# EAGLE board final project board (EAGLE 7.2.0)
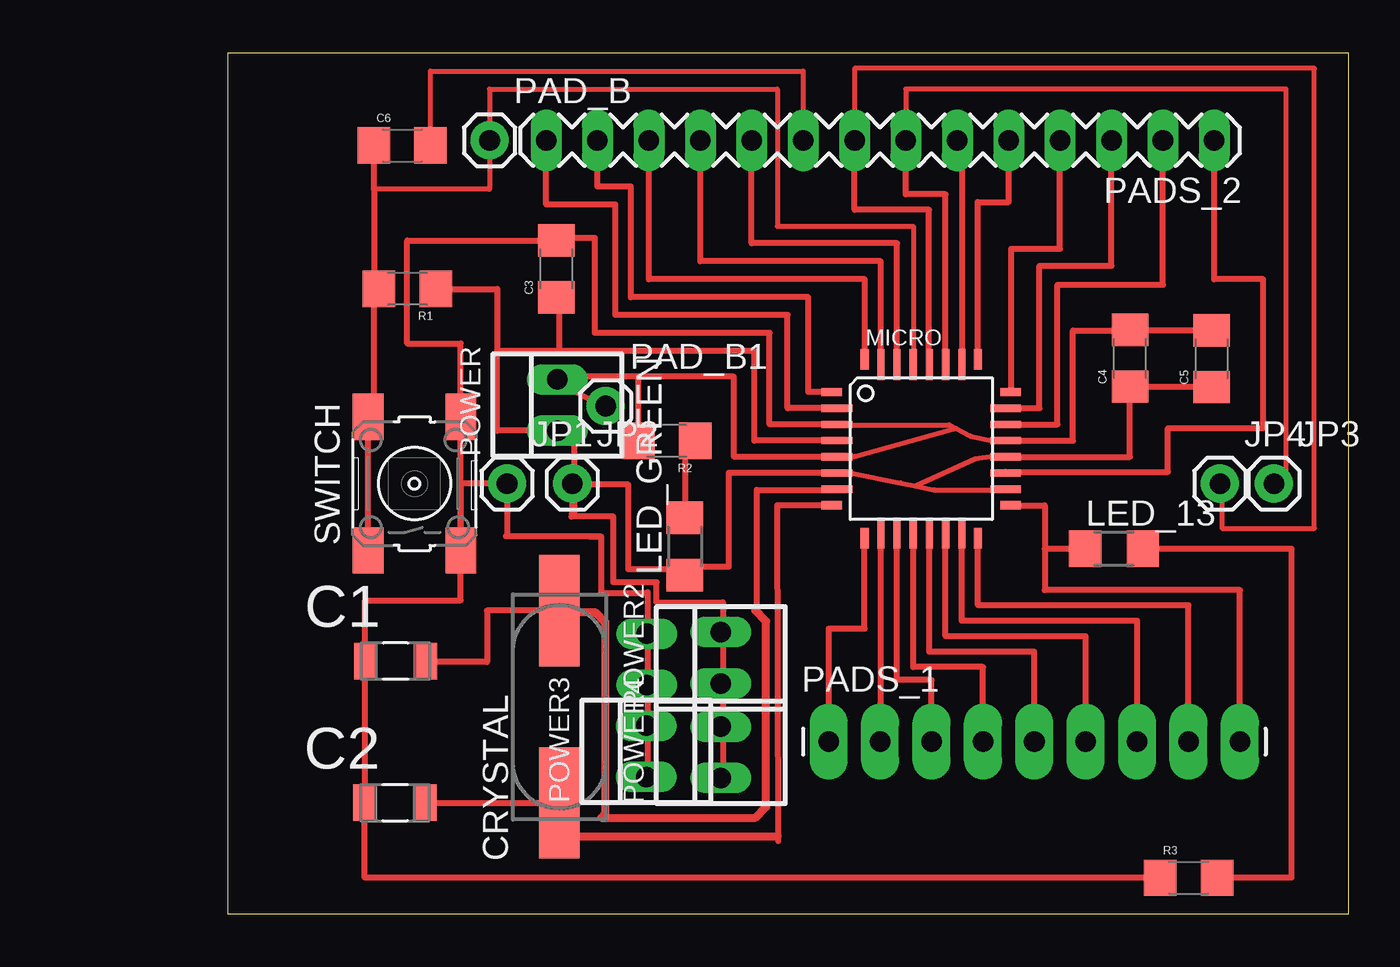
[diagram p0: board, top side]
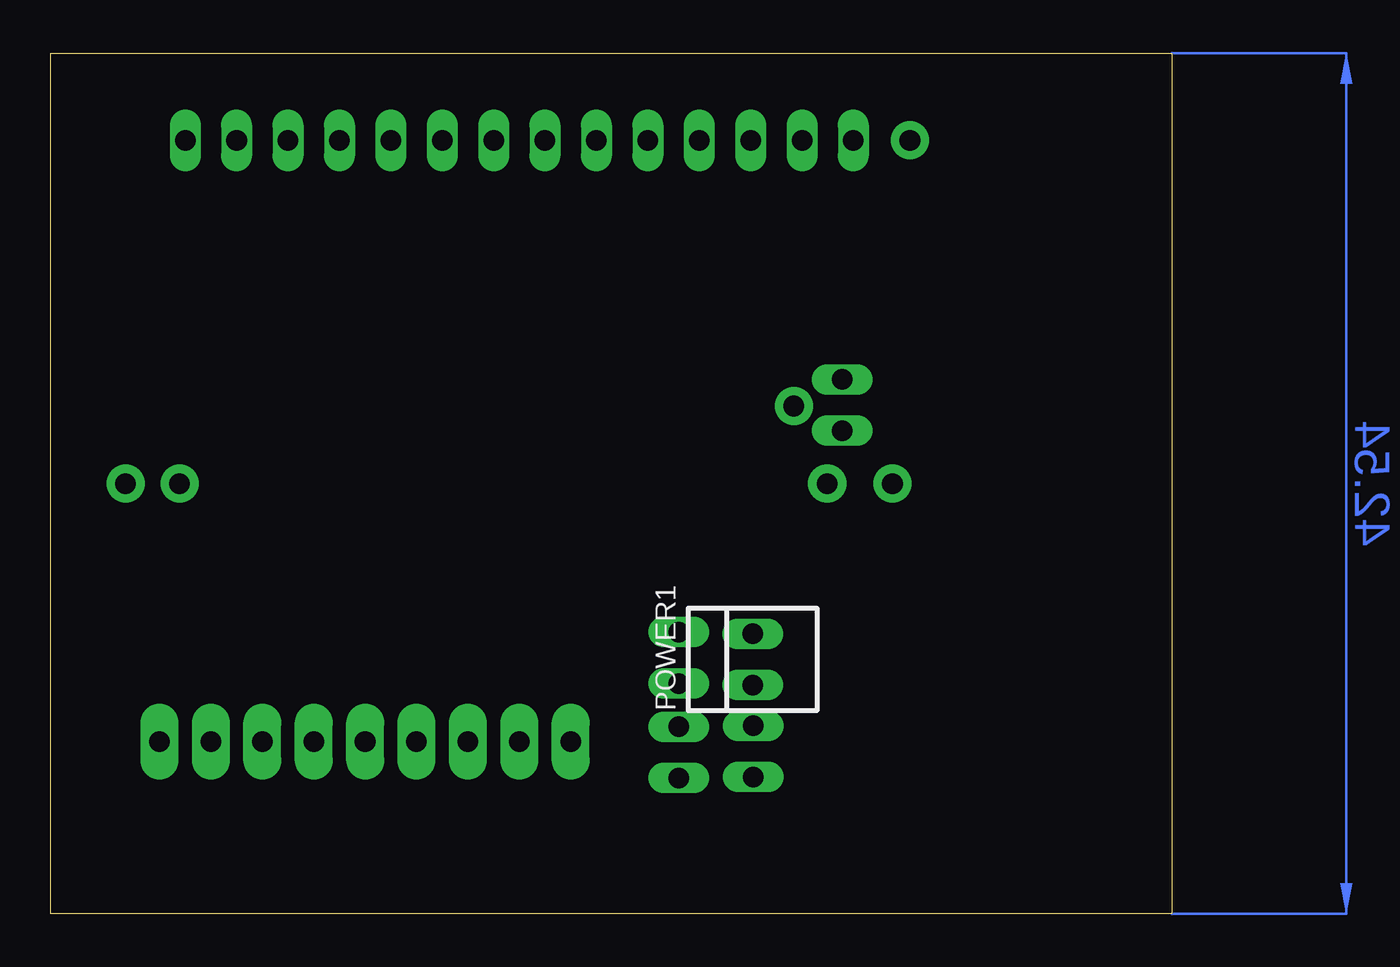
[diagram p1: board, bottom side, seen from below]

Size 55.42 x 42.54 mm. Coordinates in mm from the lower left corner, seen from the top.
Outline: 0,0 55.42,0 55.42,42.54 0,42.54 0,0
Copper layers (1*16): Top 0.035mm / dielectric 1.5mm / Bottom 0.035mm
Design rules "default": minimum track width 10mil, minimum drill 24mil, track to track 8mil, track to pad 8mil, pad to pad 8mil, via to via 8mil, smd to smd 8mil, copper to edge 40mil, drill to drill 8mil, minimum pad ring 10mil, minimum via ring 8mil, stop-mask expansion 4mil, vias tented up to drill 0mil, thermal gap 10mil

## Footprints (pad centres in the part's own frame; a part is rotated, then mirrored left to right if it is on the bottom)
CAPC3216X178N = smd 1.118 x 1.803: 1 -1.499,0; 2 1.499,0
1206 = smd 1.6 x 1.8: 1 -1.4,0; 2 1.4,0
CSM-7X-DU = smd 5.5 x 2: 1 -4.75,0; 2 4.75,0
1X01 = drill 1.016 pad 1.88: 1 0,0
1206' = smd 1.6 x 1.803: 1 -1.422,0; 2 1.422,0
TQFP32-08 = smd 1.016 x 0.406: 1 -4.42,2.8; 8 -4.42,-2.8; 17 4.42,-2.8; 24 4.42,2.8 | smd 1.524 x 0.356: 2 -4.166,2; 3 -4.166,1.2; 4 -4.166,0.4; 5 -4.166,-0.4; 6 -4.166,-1.2; 7 -4.166,-2; 18 4.166,-2; 19 4.166,-1.2; 20 4.166,-0.4; 21 4.166,0.4; 22 4.166,1.2; 23 4.166,2 | smd 0.406 x 1.016: 9 -2.8,-4.42; 16 2.8,-4.42; 25 2.8,4.42; 32 -2.8,4.42 | smd 0.356 x 1.524: 10 -2,-4.166; 11 -1.2,-4.166; 12 -0.4,-4.166; 13 0.4,-4.166; 14 1.2,-4.166; 15 2,-4.166; 26 2,4.166; 27 1.2,4.166; 28 0.4,4.166; 29 -0.4,4.166; 30 -1.2,4.166; 31 -2,4.166
1X09_LONGPADS = drill 1.016 pad 1.88 long: 1 0,0; 2 2.54,0; 3 5.08,0; 4 7.62,0; 5 10.16,0; 6 12.7,0; 7 15.24,0; 8 17.78,0; 9 20.32,0
1X14-LONGPADS = drill 1.016 long: 1 0,0; 2 2.54,0; 3 5.08,0; 4 7.62,0; 5 10.16,0; 6 12.7,0; 7 15.24,0; 8 17.78,0; 9 20.32,0; 10 22.86,0; 11 25.4,0; 12 27.94,0; 13 30.48,0; 14 33.02,0
22-23-2021 = drill 1 long: 1 -1.27,0; 2 1.27,0
6MM_SWITCH = smd 2.286 x 1.524: 1 -3.302,2.286; 2 3.302,2.286; 3 -3.302,-2.286; 4 3.302,-2.286

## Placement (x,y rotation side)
C1  22pF  [CAPC3216X178N]  8.31,12.5 0 top
C2  22pF  [CAPC3216X178N]  8.28,5.49 0 top
C3  10uF  [1206]  16.26,31.88 90 top
C4  1uF  [1206]  44.6,27.46 90 top
C5  100nF  [1206]  48.64,27.43 90 top
C6  100nF  [1206]  8.64,37.97 0 top
CRYSTAL  16Mhz  [CSM-7X-DU]  16.41,10.24 90 top
JP1  M01PTH  [1X01]  13.82,21.26 0 top
JP2  M01PTH  [1X01]  17.04,21.26 0 top
JP3  M01PTH  [1X01]  51.71,21.26 0 top
JP4  M01PTH  [1X01]  49.05,21.26 0 top
LED_13  YELLOW  [1206']  43.81,18.03 0 top
LED_GREEN  [1206']  22.61,18.16 90 top
MICRO  ATMEGA328P-AU  [TQFP32-08]  34.29,22.99 0 top
PAD_B  M01PTH  [1X01]  12.95,38.23 0 top
PAD_B1  M01PTH  [1X01]  18.69,25.1 0 top
PADS_1  M09LONGPADS  [1X09_LONGPADS]  29.72,8.51 0 top
PADS_2  M14LONGPADS  [1X14-LONGPADS]  48.77,38.23 180 top
POWER  22-23-2021  [22-23-2021]  16.31,25.15 90 top
POWER1  22-23-2021  [22-23-2021]  20.73,12.57 90 bottom
POWER2  22-23-2021  [22-23-2021]  24.38,12.65 90 top
POWER3  22-23-2021  [22-23-2021]  20.7,8.03 90 top
POWER4  22-23-2021  [22-23-2021]  24.38,7.98 90 top
R1  10k  [1206]  8.89,30.89 180 top
R2  499  [1206]  21.72,23.37 180 top
R3  499  [1206]  47.5,1.78 0 top
SWITCH  [6MM_SWITCH]  9.25,21.26 90 top

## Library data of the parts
C1 C2 = AVX_By_element14_Batch_1; MPN: 0612ZC225MAT2A; OC_FARNELL: -; OC_NEWARK: 12N3209; SUPPLIER: AVX; TOLERANCE: ±20%; VOLTAGERATING: 10V
C3-C6 JP1-JP4 PAD_B PAD_B1 PADS_1 PADS_2 R1-R3 = 01_SparkFun
CRYSTAL = 01_FAB_Hello; OC_FARNELL: unknown; OC_NEWARK: unknown
LED_13 LED_GREEN SWITCH = 01_FAB_Hello
MICRO = atmega8
POWER POWER1-POWER4 = con-molex; MF: MOLEX; MPN: 22-23-2021; OC_FARNELL: 1462926; OC_NEWARK: 25C3832

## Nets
GND: C1.1 C2.1 C3.2 C4.2 C5.2 JP1.1 MICRO.3 MICRO.5 MICRO.21 POWER.2 R2.2 R3.1 SWITCH.3 SWITCH.4
N$1: MICRO.9 PADS_1.1
N$2: MICRO.7
N$3: C6.2 PADS_2.9
N$4: MICRO.10 PADS_1.2
N$5: MICRO.11 PADS_1.3
N$6: MICRO.12 PADS_1.4
N$7: MICRO.13 PADS_1.5
N$8: MICRO.14 PADS_1.6
N$9: MICRO.8
N$10: MICRO.15 PADS_1.7
N$11: MICRO.16 PADS_1.8
N$12: LED_13.1 MICRO.17 PADS_1.9
N$13: MICRO.19 PADS_2.1
N$14: MICRO.22 PADS_2.2
N$15: MICRO.23 PADS_2.3
N$16: MICRO.24 PADS_2.4
N$17: MICRO.25 PADS_2.5
N$18: MICRO.26 PADS_2.6
N$19: JP3.1 MICRO.27 PADS_2.7
N$20: MICRO.30 PADS_2.10
N$21: MICRO.31 PADS_2.11
N$22: MICRO.32 PADS_2.12
N$23: MICRO.1 PADS_2.13
N$24: MICRO.2 PADS_2.14
N$25: JP4.1 MICRO.28 PADS_2.8
N$26: LED_GREEN.2 R2.1
N$27: LED_13.2 R3.2
N$28: C6.1 MICRO.29 PAD_B.1 R1.2 SWITCH.1 SWITCH.2
S$1: C2.2 CRYSTAL.1
S$3: C1.2 CRYSTAL.2
VCC: C3.1 C4.1 C5.1 JP2.1 LED_GREEN.1 MICRO.4 MICRO.6 MICRO.18 MICRO.20 POWER.1 R1.1

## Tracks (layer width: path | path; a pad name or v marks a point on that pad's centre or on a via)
GND
  Top 0.254: MICRO.3 30.15,24.16 35.68,24.16 | 35.68,24.16 36.7,23.62 37.85,23.37 | 30.73,22.61 30.99,22.61 35.86,23.95 | 35.86,23.95 36,23.99 | 35.68,24.16 35.86,23.95
  Top 0.305: MICRO.5 | MICRO.21 | 6.68,5.49 C2.1 6.78,1.78 R3.1 | 20.83,23.88 R2.2 20.83,24.13 | 20.83,23.88 | MICRO.5 30.12,22.61 25.02,22.61 25.02,26.54 20.32,26.54 | 30.73,22.61 MICRO.5 | MICRO.21 37.85,23.37 | MICRO.3 26.8,24.19 26.8,28.7 18.16,28.7 18.16,33.4 16.26,33.4 C3.2 8.89,33.27 8.89,28.19 11.53,28.19 SWITCH.4 SWITCH.3 | 6.73,5.97 6.81,5.97 C1.1 | C1.1 6.73,12.5 | 20.32,26.54 16.31,26.54 POWER.2 | 20.83,23.88 20.32,23.88 | 20.32,23.88 20.32,26.54 | 6.86,12.5 C1.1 | C1.1 6.81,15.49 11.53,15.49 SWITCH.3 | JP1.1 11.53,21.26 SWITCH.3 | MICRO.21 41.78,23.39 41.78,28.83 44.6,28.83 C4.2 48.64,28.86 C5.2 | 20.32,23.88 20.19,23.88
  Top 0.406: C2.1 6.73,5.49 | 6.73,5.49 6.73,5.46 | 6.73,5.49 6.73,5.97
N$1
  Top 0.305: PADS_1.1 29.72,14.1 31.49,14.1 MICRO.9
N$2
  Top 0.305: 26.16,14.99 26.16,20.95 30.12,20.95 MICRO.7
N$3
  Top 0.254: C6.2 10.03,41.66 28.45,41.66 PADS_2.9
N$4
  Top 0.305: PADS_1.2 32.29,8.51 MICRO.10
N$5
  Top 0.305: PADS_1.3 34.8,11.56 33.09,11.56 MICRO.11
N$6
  Top 0.305: 33.91,18.82 MICRO.12 33.89,12.19 37.34,12.19 PADS_1.4
N$7
  Top 0.305: MICRO.13 34.69,12.95 39.88,12.95 PADS_1.5
N$8
  Top 0.305: MICRO.14 35.49,13.72 42.42,13.72 PADS_1.6
N$9
  Top 0.305: 27.23,3.58 27.18,20.19 MICRO.8
N$10
  Top 0.305: PADS_1.7 44.96,14.48 36.29,14.48 MICRO.15
N$11
  Top 0.305: MICRO.16 37.09,15.24 47.5,15.24 PADS_1.8
N$12
  Top 0.305: 40.39,18.03 40.39,16 50.04,16 PADS_1.9 | LED_13.1 40.39,18.03 | MICRO.17 40.39,20.19 40.39,18.03
N$13
  Top 0.305: MICRO.19 38.46,21.84 46.48,21.84 46.48,24 51.18,24 51.18,31.37 48.77,31.37 PADS_2.1
N$14
  Top 0.305: MICRO.22 41.02,24.19 41.02,31.09 46.23,31.09 PADS_2.2
N$15
  Top 0.305: MICRO.23 40.13,24.99 40.13,32.03 43.69,32.03 PADS_2.3
N$16
  Top 0.305: PADS_2.4 41.15,32.87 38.73,32.87 38.73,25.79 MICRO.24
N$17
  Top 0.305: MICRO.25 37.08,35.18 38.61,35.18 PADS_2.5
N$18
  Top 0.305: MICRO.26 36.32,27.15 36.32,37.34 arc-90 36.07,37.59 PADS_2.6
N$19
  Top 0.254: PADS_2.7 33.53,40.77 52.32,40.77 52.32,21.29 51.71,21.29 JP3.1
  Top 0.305: MICRO.27 35.49,35.56 33.53,35.56 PADS_2.7
N$20
  Top 0.305: MICRO.30 33.09,33.15 25.91,33.15 PADS_2.10
N$21
  Top 0.305: MICRO.31 32.29,32.26 23.37,32.26 PADS_2.11
N$22
  Top 0.305: PADS_2.12 20.83,31.37 31.5,31.37 MICRO.32
N$23
  Top 0.305: MICRO.1 28.7,25.79 28.7,30.48 19.94,30.48 19.94,35.94 18.29,35.94 PADS_2.13
N$24
  Top 0.305: MICRO.2 27.69,24.99 27.69,29.59 19.18,29.59 19.18,35.05 15.75,35.05 PADS_2.14
N$25
  Top 0.254: JP4.1 49.15,21.26 49.15,19.05 53.72,19.05 53.72,41.78 30.99,41.78 PADS_2.8
  Top 0.305: MICRO.28 34.67,27.15 34.67,34.8 30.99,34.8 PADS_2.8
N$26
  Top 0.305: 23.49,23.75 R2.1 22.61,23.62 LED_GREEN.2
N$27
  Top 0.305: LED_13.2 52.58,18.03 52.58,1.78 R3.2
N$28
  Top 0.254: MICRO.29 33.89,33.98 27.18,33.98 27.18,40.77 12.95,40.77 PAD_B.1 12.95,35.81 7.24,35.81
  Top 0.305: C6.1 7.24,35.81 7.24,31.5 | 7.24,31.5 7.49,31.5 R1.2 | SWITCH.1 SWITCH.2 7.49,24.64 7.24,24.64 7.24,31.5
S$1
  Top 0.305: C2.2 CRYSTAL.1 | 9.78,5.46 C2.2 | C2.2
S$2
  Top 0.406: 16.92,3.83 27.2,3.83
S$3
  Top 0.305: CRYSTAL.2 12.83,14.99 12.83,12.45 9.8,12.45 C1.2
S$4
  Top 0.406: 16.79,14.91 18.16,14.91 18.67,14.4 18.67,4.95 18.47,4.75 26.09,4.75 26.62,5.28 26.62,14.45 26.09,14.99
S$5
  Top 0.305: 21.23,15.39 24.49,15.39 24.49,6.71
S$6
  Top 0.305: 13.82,21.21 13.82,18.72
S$7
  Top 0.305: 17.91,18.64 18.47,18.64 18.47,15.85 20.55,15.85
S$8
  Top 0.305: 16.2,26.31 18.77,24.99
S$9
  Top 0.305: 13.77,18.67 18.41,18.67
S$10
  Top 0.305: 21.21,15.37 21.21,16.38 19.08,16.38 19.08,19.63 16.99,19.63
S$11
  Top 0.305: 20.78,6.83 20.78,15.9 20.5,15.82
VCC
  Top 0.254: 30.81,21.79 33.27,21.29 34.02,21.14 | 34.02,21.14 34.92,20.95 38.46,20.95 | MICRO.20 37.85,22.59 37.85,22.61 36.96,22.48 34.02,21.14
  Top 0.305: MICRO.18 38.46,20.95 | MICRO.20 | MICRO.4 26.03,23.39 26.03,27.81 16.38,27.81 | 16.38,27.81 13.34,27.81 | LED_GREEN.1 22.61,17.14 22.73,17.14 | MICRO.20 37.85,22.61 | 30.81,21.79 MICRO.6 24.77,21.79 24.77,17.14 22.73,17.14 | R1.1 13.34,30.89 13.34,27.81 | C3.1 16.38,30.48 16.38,27.81 | 13.34,27.81 13.34,23.88 POWER.1 17.14,23.88 | 17.14,23.88 17.27,23.88 | 17.27,21.21 JP2.1 17.04,21.21 17.07,21.21 17.14,21.21 | 22.73,17.14 22.73,17.02 19.81,17.02 19.81,21.21 17.14,21.21 | 17.14,21.21 17.14,23.88 | MICRO.20 44.6,22.59 C4.1 48.64,26.06 C5.1
  Top 0.406: 17.07,21.21 17.07,19.74
(copper drawn outside any net)
  shapes: Bottom area x1

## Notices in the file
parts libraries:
01_SparkFun: Licensing: CC v3.0 Share-Alike You are welcome to use this library for commercial purposes.
